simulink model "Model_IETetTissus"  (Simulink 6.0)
settings: Solver=ode45  StartTime=0  StopTime=7E-3  RelTol=1e-3
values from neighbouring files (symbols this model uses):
  b = S/Sm    (= 0.1)    [Constantes.m]    (also in ConstantesBck.m)
  beta = 0.95    [Constantes.m]    (also in ConstantesBck.m; ResCourV1.m = 1; ResCrV1.m = 1; ResEnerV1.m = 1)
  C = 1    [Constantes.m]    (also in ConstantesBck.m)
  Cdl = 603E-9    (= 6.03e-07)    [Constantes.m]    (also in ConstantesBck.m; ResCourV1.m = 7.313e-07; ResCrV1.m = 7.313e-07; ResEnerV1.m = 7.313e-07)
  Cmem = 1E-6*Sm*(1-b)    (= 2.826e-08)    [Constantes.m]    (also in ConstantesBck.m = 3.14e-11; ImpedanceZtissus.m = 4e-08; Ztissus.m = 4e-08; CalculCharge.m = 1)
  gk = 36    [Constantes.m]    (also in ConstantesBck.m; sim_hh.m)
  gl = 0.3    [Constantes.m]    (also in ConstantesBck.m; sim_hh.m)
  gna = 120    [Constantes.m]    (also in ConstantesBck.m; sim_hh.m)
  h0 = 0.5961    [Constantes.m]    (also in ConstantesBck.m)
  m0 = 0.0529    [Constantes.m]    (also in ConstantesBck.m)
  mK = 0    [Constantes.m]    (also in ConstantesBck.m)
  mL = 0    [Constantes.m]    (also in ConstantesBck.m)
  mNa = 0    [Constantes.m]    (also in ConstantesBck.m)
  n0 = 0.3177    [Constantes.m]    (also in ConstantesBck.m)
  rapportIE = 10    [Constantes.m]
  Rcan = 6.398E3*Sm*(1-b)    (= 180.80748)    [Constantes.m]    (also in ConstantesBck.m = 0.03454; ImpedanceZtissus.m = 44; Ztissus.m = 44)
  Rct = 185.6E3    (= 185600)    [Constantes.m]    (also in ConstantesBck.m; ResCourV1.m = 605200; ResCrV1.m = 605200; ResEnerV1.m = 605200)
  Rext = 2.9E3    (= 2900)    [Constantes.m]    (also in ConstantesBck.m)
  Rint = 2.9E2    (= 290)    [Constantes.m]    (also in ConstantesBck.m = 400)
  sigma = 66466    [Constantes.m]    (also in ConstantesBck.m; ResCourV1.m = 68000; ResCrV1.m = 68000; ResEnerV1.m = 68000)
  Sm = 3.14e-2    (= 0.0314)    [Constantes.m]    (also in ConstantesBck.m = 0.000314)
  t0 = 2E-3    (= 0.002)    [Constantes.m]    (also in ConstantesBck.m = 0.001)
  Vk = -82    [Constantes.m]    (also in ConstantesBck.m)
  Vl = -59    [Constantes.m]    (also in ConstantesBck.m)
  Vna = 45    [Constantes.m]    (also in ConstantesBck.m)
  Vr = -70    [Constantes.m]    (also in ConstantesBck.m)
undefined symbols (not defined in the file or in its folder): ln

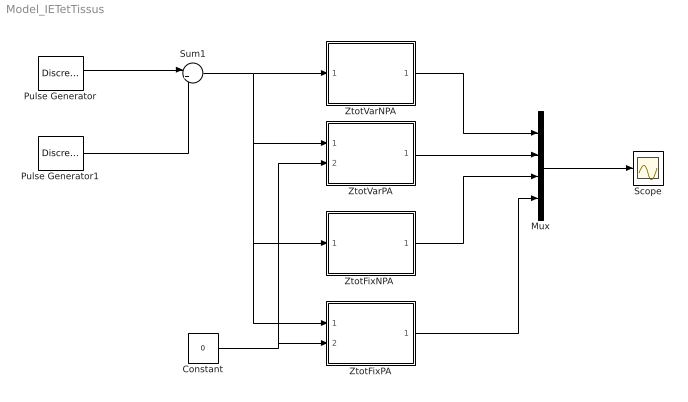
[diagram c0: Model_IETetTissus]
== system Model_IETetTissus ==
  Constant : Constant  Value=0
  Mux : Mux
  Pulse Generator : DiscretePulseGenerator  PulseType=Time based  Amplitude=-160E-6  Period=2*t0  PulseWidth=50  PhaseDelay=t0
  Pulse Generator1 : DiscretePulseGenerator  PulseType=Time based  Amplitude=160E-6  Period=2*t0  PulseWidth=50  PhaseDelay=2*t0
  Scope : Scope
  Sum1 : Sum  Inputs=|++
  "ZtotFixNPA " : Subsystem
  ZtotFixPA : Subsystem
  ZtotVarNPA : Subsystem
  ZtotVarPA : Subsystem
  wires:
  Pulse Generator/1 -> Sum1/1
  Pulse Generator1/1 -> Sum1/2
  Sum1/1 -> ZtotVarNPA/1(InZtot), ZtotVarPA/1(InZtot), "ZtotFixNPA "/1(InZtot), ZtotFixPA/1(InZtot)
  "ZtotFixNPA "/1(OutZtot) -> Mux/3
  ZtotVarPA/1(OutZtot) -> Mux/2
  ZtotFixPA/1(OutZtot) -> Mux/4
  Constant/1 -> ZtotFixPA/2(InVref), ZtotVarPA/2(InVref)
  ZtotVarNPA/1(OutZtot) -> Mux/1
  Mux/1 -> Scope/1

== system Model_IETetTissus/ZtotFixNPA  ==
  InZtot : Inport  Port=1  LatchInput=off
  Gain : Gain
  Sum : Sum  Inputs=|++
  Ziet : Subsystem
  Zmembrane : Subsystem
  OutZtot : Outport
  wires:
  Ziet/1(OutZiet) -> Gain/1
  Zmembrane/1(OutZmem) -> Sum/1
  InZtot/1 -> Zmembrane/1(InZmem), Ziet/1(InZiet)
  Gain/1 -> Sum/2
  Sum/1 -> OutZtot/1

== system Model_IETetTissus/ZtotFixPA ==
  InZtot : Inport  Port=1  LatchInput=off
  InVref : Inport  Port=2  LatchInput=off
  Gain : Gain
  Sum : Sum  Inputs=|++
  ZTissus : Subsystem
  Ziet : Subsystem
  OutZtot : Outport
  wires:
  ZTissus/1(Vout) -> Sum/2
  Ziet/1(OutZiet) -> Gain/1
  InZtot/1 -> ZTissus/1(IStim), Ziet/1(InZiet)
  Sum/1 -> OutZtot/1
  Gain/1 -> Sum/1
  InVref/1 -> ZTissus/2(Vref)

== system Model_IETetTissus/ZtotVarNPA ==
  InZtot : Inport  Port=1  LatchInput=off
  Gain : Gain
  Sum : Sum  Inputs=|++
  ZietVar : Subsystem
  ZmembraneVar : Subsystem
  OutZtot : Outport
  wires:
  ZietVar/1(OutZiet) -> Gain/1
  ZmembraneVar/1(OutZmem) -> Sum/1
  InZtot/1 -> ZmembraneVar/1(InZmem), ZietVar/1(InZiet)
  Gain/1 -> Sum/2
  Sum/1 -> OutZtot/1

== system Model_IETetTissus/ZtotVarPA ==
  InZtot : Inport  Port=1  LatchInput=off
  InVref : Inport  Port=2  LatchInput=off
  Gain : Gain
  Sum : Sum  Inputs=|++
  ZTissusVar : Subsystem
  ZietVar : Subsystem
  OutZtot : Outport
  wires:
  ZietVar/1(OutZiet) -> Gain/1
  ZTissusVar/1(Vout) -> Sum/1
  InZtot/1 -> ZTissusVar/1(IStim), ZietVar/1(InZiet)
  Gain/1 -> Sum/2
  Sum/1 -> OutZtot/1
  InVref/1 -> ZTissusVar/2(Vref)

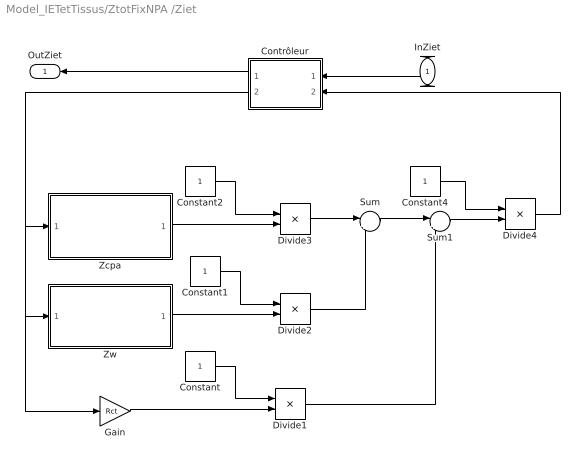
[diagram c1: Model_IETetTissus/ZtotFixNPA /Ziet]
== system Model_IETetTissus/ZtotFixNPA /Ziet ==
  InZiet : Inport  Orientation=left  Port=1  LatchInput=off
  Constant{,1..2,4} (4 alike) : Constant
  Contrôleur : Stateflow chart  Orientation=left
  Divide{1..4} (4 alike) : Product  Inputs=*/  OutScaling=2^-10
  Gain : Gain  Gain=Rct
  Sum : Sum  Inputs=|++
  Sum1 : Sum  Inputs=|++
  Zcpa : Subsystem
  Zw : Subsystem
  OutZiet : Outport  Orientation=left
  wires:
  Constant/1 -> Divide1/1
  Constant1/1 -> Divide2/1
  Constant2/1 -> Divide3/1
  Zcpa/1(OutZcpa) -> Divide3/2
  Zw/1(OutZw) -> Divide2/2
  Divide3/1 -> Sum/1
  Constant4/1 -> Divide4/1
  Divide2/1 -> Sum/2
  Sum/1 -> Sum1/1
  Divide1/1 -> Sum1/2
  Sum1/1 -> Divide4/2
  Divide4/1 -> Contrôleur/2(calc)
  Gain/1 -> Divide1/2
  InZiet/1 -> Contrôleur/1(u)
  Contrôleur/1(y) -> OutZiet/1
  Contrôleur/2(temp) -> Zcpa/1(InZcpa), Zw/1(InZw), Gain/1

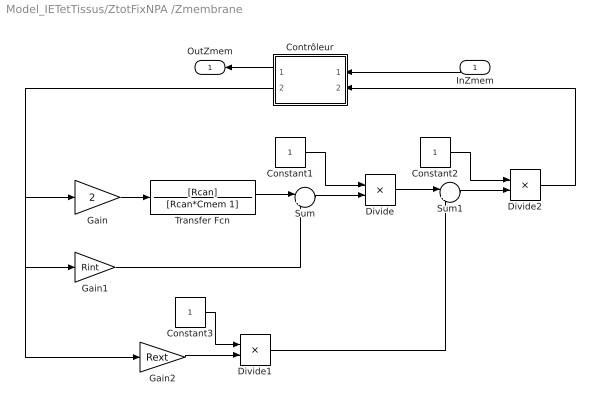
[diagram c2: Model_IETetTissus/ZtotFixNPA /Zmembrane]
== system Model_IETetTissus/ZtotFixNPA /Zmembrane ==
  InZmem : Inport  Orientation=left  Port=1  LatchInput=off
  Constant1 : Constant
  Constant2 : Constant
  Constant3 : Constant
  Contrôleur : Stateflow chart  Orientation=left
  Divide : Product  Inputs=*/  OutScaling=2^-10
  Divide1 : Product  Inputs=*/  OutScaling=2^-10
  Divide2 : Product  Inputs=*/  OutScaling=2^-10
  Gain : Gain  Gain=2
  Gain1 : Gain  Gain=Rint
  Gain2 : Gain  Gain=Rext
  Sum : Sum  Inputs=|++
  Sum1 : Sum  Inputs=|++
  Transfer Fcn : TransferFcn  Numerator=[Rcan]  Denominator=[Rcan*Cmem 1]
  OutZmem : Outport  Orientation=left
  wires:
  Gain/1 -> Transfer Fcn/1
  Transfer Fcn/1 -> Sum/1
  Sum/1 -> Divide/2
  Gain2/1 -> Divide1/2
  Constant1/1 -> Divide/1
  Divide/1 -> Sum1/1
  Constant2/1 -> Divide2/1
  Sum1/1 -> Divide2/2
  Gain1/1 -> Sum/2
  Divide1/1 -> Sum1/2
  Divide2/1 -> Contrôleur/2(calc)
  Constant3/1 -> Divide1/1
  Contrôleur/2(temp) -> Gain2/1, Gain1/1, Gain/1
  InZmem/1 -> Contrôleur/1(u)
  Contrôleur/1(y) -> OutZmem/1

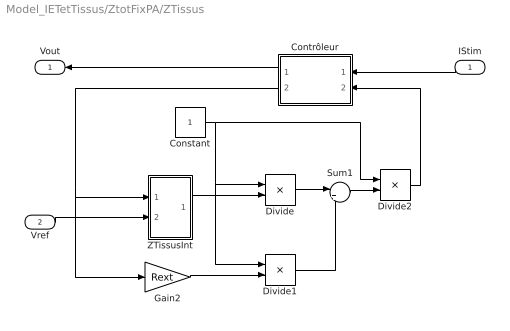
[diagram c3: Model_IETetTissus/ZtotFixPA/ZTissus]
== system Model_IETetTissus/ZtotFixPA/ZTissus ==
  IStim : Inport  Orientation=left  Port=1  LatchInput=off
  Vref : Inport  Port=2  LatchInput=off
  Constant : Constant
  Contrôleur : Stateflow chart  Orientation=left
  Divide : Product  Inputs=*/  OutScaling=2^-10
  Divide1 : Product  Inputs=*/  OutScaling=2^-10
  Divide2 : Product  Inputs=*/  OutScaling=2^-10
  Gain2 : Gain  Gain=Rext
  Sum1 : Sum  Inputs=|++
  ZTissusInt : Subsystem
  Vout : Outport  Orientation=left
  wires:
  Constant/1 -> Divide/1, Divide1/1, Divide2/1
  ZTissusInt/1(Vout) -> Divide/2
  Gain2/1 -> Divide1/2
  Divide/1 -> Sum1/1
  Divide1/1 -> Sum1/2
  Sum1/1 -> Divide2/2
  Vref/1 -> ZTissusInt/2(VRefIn)
  Divide2/1 -> Contrôleur/2(calc)
  Contrôleur/2(temp) -> ZTissusInt/1(InStim), Gain2/1
  IStim/1 -> Contrôleur/1(u)
  Contrôleur/1(y) -> Vout/1

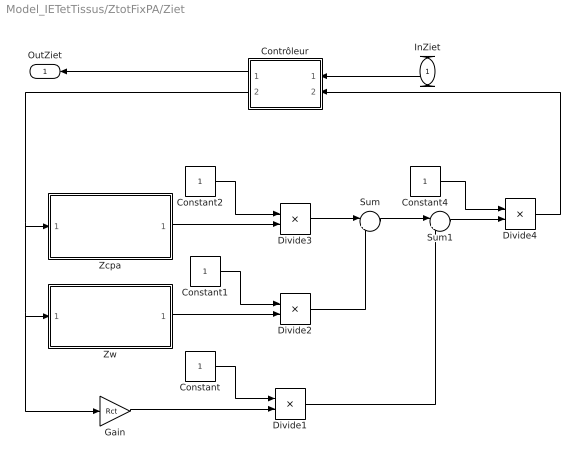
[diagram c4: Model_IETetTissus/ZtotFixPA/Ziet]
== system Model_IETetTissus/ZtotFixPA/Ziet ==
  InZiet : Inport  Orientation=left  Port=1  LatchInput=off
  Constant{,1..2,4} (4 alike) : Constant
  Contrôleur : Stateflow chart  Orientation=left
  Divide{1..4} (4 alike) : Product  Inputs=*/  OutScaling=2^-10
  Gain : Gain  Gain=Rct
  Sum : Sum  Inputs=|++
  Sum1 : Sum  Inputs=|++
  Zcpa : Subsystem
  Zw : Subsystem
  OutZiet : Outport  Orientation=left
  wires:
  Constant/1 -> Divide1/1
  Constant1/1 -> Divide2/1
  Constant2/1 -> Divide3/1
  Zcpa/1(OutZcpa) -> Divide3/2
  Zw/1(OutZw) -> Divide2/2
  Divide3/1 -> Sum/1
  Constant4/1 -> Divide4/1
  Divide2/1 -> Sum/2
  Sum/1 -> Sum1/1
  Divide1/1 -> Sum1/2
  Sum1/1 -> Divide4/2
  Divide4/1 -> Contrôleur/2(calc)
  Gain/1 -> Divide1/2
  InZiet/1 -> Contrôleur/1(u)
  Contrôleur/1(y) -> OutZiet/1
  Contrôleur/2(temp) -> Zcpa/1(InZcpa), Zw/1(InZw), Gain/1

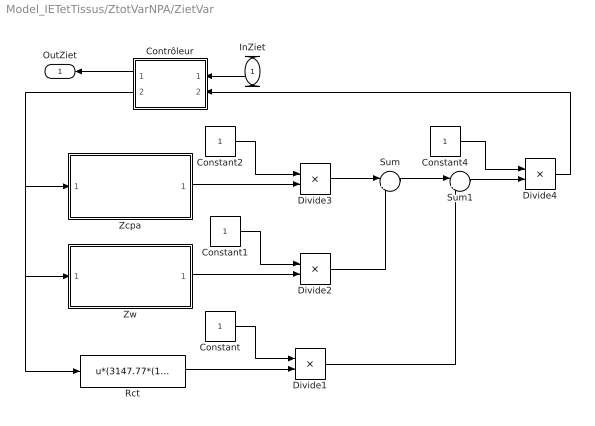
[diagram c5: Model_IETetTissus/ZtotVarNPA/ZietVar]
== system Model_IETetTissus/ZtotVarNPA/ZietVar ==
  InZiet : Inport  Orientation=left  Port=1  LatchInput=off
  Constant{,1..2,4} (4 alike) : Constant
  Contrôleur : Stateflow chart  Orientation=left
  Divide{1..4} (4 alike) : Product  Inputs=*/  OutScaling=2^-10
  Rct : Fcn  Expr=u*(3147.77*(1/((1E6*abs(u))^0.7199)))*1000
  Sum : Sum  Inputs=|++
  Sum1 : Sum  Inputs=|++
  Zcpa : Subsystem
  Zw : Subsystem
  OutZiet : Outport  Orientation=left
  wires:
  Constant/1 -> Divide1/1
  Constant1/1 -> Divide2/1
  Constant2/1 -> Divide3/1
  Zcpa/1(OutZcpa) -> Divide3/2
  Zw/1(OutZw) -> Divide2/2
  Rct/1 -> Divide1/2
  Divide3/1 -> Sum/1
  Constant4/1 -> Divide4/1
  Divide2/1 -> Sum/2
  Sum/1 -> Sum1/1
  Divide1/1 -> Sum1/2
  Sum1/1 -> Divide4/2
  Contrôleur/2(temp) -> Rct/1, Zw/1(InZw), Zcpa/1(InZcpa)
  InZiet/1 -> Contrôleur/1(u)
  Contrôleur/1(y) -> OutZiet/1
  Divide4/1 -> Contrôleur/2(calc)

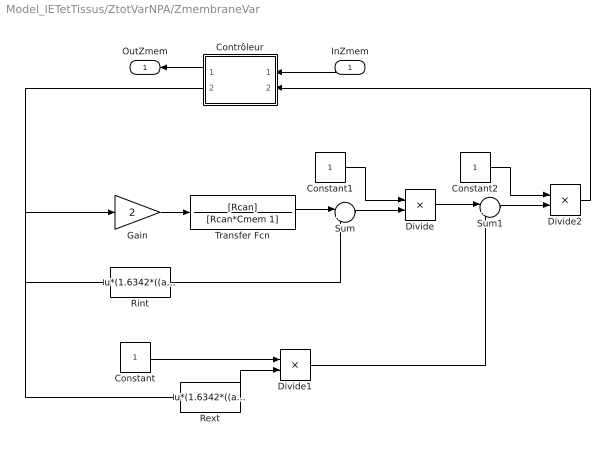
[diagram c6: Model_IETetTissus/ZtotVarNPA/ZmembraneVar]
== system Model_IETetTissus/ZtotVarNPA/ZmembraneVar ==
  InZmem : Inport  Orientation=left  Port=1  LatchInput=off
  Constant : Constant
  Constant1 : Constant
  Constant2 : Constant
  Contrôleur : Stateflow chart  Orientation=left
  Divide : Product  Inputs=*/  OutScaling=2^-10
  Divide1 : Product  Inputs=*/  OutScaling=2^-10
  Divide2 : Product  Inputs=*/  OutScaling=2^-10
  Gain : Gain  Gain=2
  Rext : Fcn  Expr=u*(1.6342*((abs(u)*1E6)^0.1267))*1E3
  Rint : Fcn  Expr=u*(1.6342*((abs(u)*1E6)^0.1267))*1E3/rapportIE
  Sum : Sum  Inputs=|++
  Sum1 : Sum  Inputs=|++
  Transfer Fcn : TransferFcn  Numerator=[Rcan]  Denominator=[Rcan*Cmem 1]
  OutZmem : Outport  Orientation=left
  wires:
  Gain/1 -> Transfer Fcn/1
  Transfer Fcn/1 -> Sum/1
  Sum/1 -> Divide/2
  Rext/1 -> Divide1/2
  Constant1/1 -> Divide/1
  Constant/1 -> Divide1/1
  Divide/1 -> Sum1/1
  Constant2/1 -> Divide2/1
  Sum1/1 -> Divide2/2
  Rint/1 -> Sum/2
  Divide1/1 -> Sum1/2
  Contrôleur/2(temp) -> Rext/1, Rint/1, Gain/1
  Divide2/1 -> Contrôleur/2(calc)
  InZmem/1 -> Contrôleur/1(u)
  Contrôleur/1(y) -> OutZmem/1

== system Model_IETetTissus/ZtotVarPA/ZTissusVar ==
  IStim : Inport  Orientation=left  Port=1  LatchInput=off
  Vref : Inport  Port=2  LatchInput=off
  Constant : Constant
  Contrôleur : Stateflow chart  Orientation=left
  Divide : Product  Inputs=*/  OutScaling=2^-10
  Divide1 : Product  Inputs=*/  OutScaling=2^-10
  Divide2 : Product  Inputs=*/  OutScaling=2^-10
  Rext1 : Fcn  Expr=u*(1.6342*((abs(u)*1E6)^0.1267))*1E3
  Sum1 : Sum  Inputs=|++
  ZTissusInt : Subsystem
  Vout : Outport  Orientation=left
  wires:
  Constant/1 -> Divide/1, Divide1/1, Divide2/1
  ZTissusInt/1(Vout) -> Divide/2
  Rext1/1 -> Divide1/2
  Divide/1 -> Sum1/1
  Divide1/1 -> Sum1/2
  Sum1/1 -> Divide2/2
  Vref/1 -> ZTissusInt/2(VRefIn)
  Divide2/1 -> Contrôleur/2(calc)
  Contrôleur/2(temp) -> Rext1/1, ZTissusInt/1(InStim)
  IStim/1 -> Contrôleur/1(u)
  Contrôleur/1(y) -> Vout/1

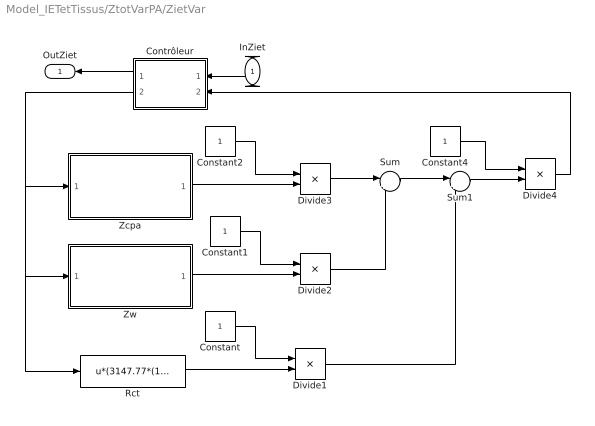
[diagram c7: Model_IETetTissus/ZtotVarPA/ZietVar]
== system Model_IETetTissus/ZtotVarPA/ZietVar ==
  InZiet : Inport  Orientation=left  Port=1  LatchInput=off
  Constant{,1..2,4} (4 alike) : Constant
  Contrôleur : Stateflow chart  Orientation=left
  Divide{1..4} (4 alike) : Product  Inputs=*/  OutScaling=2^-10
  Rct : Fcn  Expr=u*(3147.77*(1/((1E6*abs(u))^0.7199)))*1000
  Sum : Sum  Inputs=|++
  Sum1 : Sum  Inputs=|++
  Zcpa : Subsystem
  Zw : Subsystem
  OutZiet : Outport  Orientation=left
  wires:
  Constant/1 -> Divide1/1
  Constant1/1 -> Divide2/1
  Constant2/1 -> Divide3/1
  Zcpa/1(OutZcpa) -> Divide3/2
  Zw/1(OutZw) -> Divide2/2
  Rct/1 -> Divide1/2
  Divide3/1 -> Sum/1
  Constant4/1 -> Divide4/1
  Divide2/1 -> Sum/2
  Sum/1 -> Sum1/1
  Divide1/1 -> Sum1/2
  Sum1/1 -> Divide4/2
  Contrôleur/2(temp) -> Rct/1, Zw/1(InZw), Zcpa/1(InZcpa)
  InZiet/1 -> Contrôleur/1(u)
  Contrôleur/1(y) -> OutZiet/1
  Divide4/1 -> Contrôleur/2(calc)

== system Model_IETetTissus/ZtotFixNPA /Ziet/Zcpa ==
  InZcpa : Inport  Port=1  LatchInput=off
  Fcn : Fcn  Expr=u^beta
  Transfer Fcn : TransferFcn  Denominator=[Cdl 0]
  OutZcpa : Outport
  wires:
  Transfer Fcn/1 -> Fcn/1
  InZcpa/1 -> Transfer Fcn/1
  Fcn/1 -> OutZcpa/1

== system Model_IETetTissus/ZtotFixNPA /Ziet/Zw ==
  InZw : Inport  Port=1  LatchInput=off
  Gain : Gain  Gain=sigma
  Math Function : Math  Operator=sqrt
  Transfer Fcn : TransferFcn  Numerator=[2]  Denominator=[1 0]
  OutZw : Outport
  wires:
  Transfer Fcn/1 -> Math Function/1
  Math Function/1 -> Gain/1
  Gain/1 -> OutZw/1
  InZw/1 -> Transfer Fcn/1

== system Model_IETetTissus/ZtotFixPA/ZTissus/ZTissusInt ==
  InStim : Inport  Orientation=down  Port=1  LatchInput=off
  VRefIn : Inport  Port=2  LatchInput=off
  Constant : Constant  Value=0
  Gain1 : Gain  Gain=Rint
  Gain2 : Gain  Gain=-1
  Gain3 : Gain  Gain=-1
  Gain4 : Gain  Gain=-1
  Modele HH : Subsystem
  Modele HH1 : Subsystem
  Sum1 : Sum  Inputs=|+++
  Vout : Outport
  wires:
  Modele HH1/1(HHout) -> Gain3/1
  Modele HH/1(HHout) -> Gain4/1
  Gain1/1 -> Sum1/2
  Gain2/1 -> Modele HH/1(HHin)
  InStim/1 -> Gain2/1, Gain1/1, Modele HH1/1(HHin)
  Constant/1 -> Modele HH1/2(VRefIn)
  Sum1/1 -> Vout/1
  VRefIn/1 -> Modele HH/2(VRefIn)
  Gain3/1 -> Sum1/1
  Gain4/1 -> Sum1/3

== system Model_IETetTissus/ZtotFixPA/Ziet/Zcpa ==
  InZcpa : Inport  Port=1  LatchInput=off
  Fcn : Fcn  Expr=u^beta
  Transfer Fcn : TransferFcn  Denominator=[Cdl 0]
  OutZcpa : Outport
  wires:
  Transfer Fcn/1 -> Fcn/1
  InZcpa/1 -> Transfer Fcn/1
  Fcn/1 -> OutZcpa/1

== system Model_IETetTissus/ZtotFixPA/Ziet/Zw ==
  InZw : Inport  Port=1  LatchInput=off
  Gain : Gain  Gain=sigma
  Math Function : Math  Operator=sqrt
  Transfer Fcn : TransferFcn  Numerator=[2]  Denominator=[1 0]
  OutZw : Outport
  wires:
  Transfer Fcn/1 -> Math Function/1
  Math Function/1 -> Gain/1
  Gain/1 -> OutZw/1
  InZw/1 -> Transfer Fcn/1

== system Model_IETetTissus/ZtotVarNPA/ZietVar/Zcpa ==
  InZcpa : Inport  Port=1  LatchInput=off
  Cdl : Fcn  Expr=u*1E9/(918.15-80.854*ln(abs(u)*1E6))
  Fcn : Fcn  Expr=u^beta
  Transfer Fcn : TransferFcn  Denominator=[1 0]
  OutZcpa : Outport
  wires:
  Transfer Fcn/1 -> Fcn/1
  InZcpa/1 -> Cdl/1
  Fcn/1 -> OutZcpa/1
  Cdl/1 -> Transfer Fcn/1

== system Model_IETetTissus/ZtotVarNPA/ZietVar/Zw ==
  InZw : Inport  Port=1  LatchInput=off
  Math Function : Math  Operator=sqrt
  Product : Product
  Transfer Fcn : TransferFcn  Numerator=[2]  Denominator=[1 0]
  sigma : Fcn  Expr=(67202-0.0688*((1E6*abs(u))^2)-11.273*(1E6*abs(u)))
  OutZw : Outport
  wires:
  Transfer Fcn/1 -> Math Function/1
  InZw/1 -> Transfer Fcn/1, sigma/1
  Math Function/1 -> Product/1
  sigma/1 -> Product/2
  Product/1 -> OutZw/1

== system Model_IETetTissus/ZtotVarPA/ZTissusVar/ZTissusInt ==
  InStim : Inport  Orientation=down  Port=1  LatchInput=off
  VRefIn : Inport  Port=2  LatchInput=off
  Constant : Constant  Value=0
  Gain2 : Gain  Gain=-1
  Gain3 : Gain  Gain=-1
  Gain4 : Gain  Gain=-1
  Modele HH : Subsystem
  Modele HH1 : Subsystem
  Rint : Fcn  Expr=u*(1.6342*((abs(u)*1E6)^0.1267))*1E3/rapportIE
  Sum1 : Sum  Inputs=|+++
  Vout : Outport
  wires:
  Modele HH1/1(HHout) -> Gain3/1
  Modele HH/1(HHout) -> Gain4/1
  Rint/1 -> Sum1/2
  Gain2/1 -> Modele HH/1(HHin)
  InStim/1 -> Gain2/1, Rint/1, Modele HH1/1(HHin)
  Constant/1 -> Modele HH1/2(VRefIn)
  Sum1/1 -> Vout/1
  VRefIn/1 -> Modele HH/2(VRefIn)
  Gain3/1 -> Sum1/1
  Gain4/1 -> Sum1/3

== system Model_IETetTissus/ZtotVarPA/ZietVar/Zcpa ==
  InZcpa : Inport  Port=1  LatchInput=off
  Cdl : Fcn  Expr=u*1E9/(918.15-80.854*ln(abs(u)*1E6))
  Fcn : Fcn  Expr=u^beta
  Transfer Fcn : TransferFcn  Denominator=[1 0]
  OutZcpa : Outport
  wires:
  Transfer Fcn/1 -> Fcn/1
  InZcpa/1 -> Cdl/1
  Fcn/1 -> OutZcpa/1
  Cdl/1 -> Transfer Fcn/1

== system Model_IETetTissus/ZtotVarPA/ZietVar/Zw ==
  InZw : Inport  Port=1  LatchInput=off
  Math Function : Math  Operator=sqrt
  Product : Product
  Transfer Fcn : TransferFcn  Numerator=[2]  Denominator=[1 0]
  sigma : Fcn  Expr=(67202-0.0688*((1E6*abs(u))^2)-11.273*(1E6*abs(u)))
  OutZw : Outport
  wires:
  Transfer Fcn/1 -> Math Function/1
  InZw/1 -> Transfer Fcn/1, sigma/1
  Math Function/1 -> Product/1
  sigma/1 -> Product/2
  Product/1 -> OutZw/1

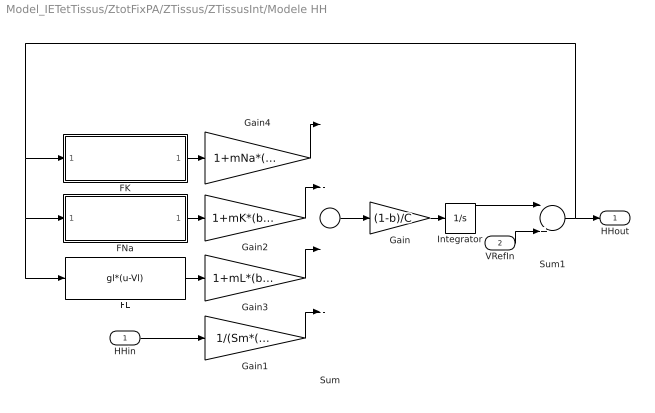
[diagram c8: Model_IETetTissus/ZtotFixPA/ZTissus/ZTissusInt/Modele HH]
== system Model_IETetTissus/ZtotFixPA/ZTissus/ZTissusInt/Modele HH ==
  HHin : Inport  Port=1  LatchInput=off
  VRefIn : Inport  Port=2  LatchInput=off
  FK : Subsystem
  FL : Fcn  Expr=gl*(u-Vl)
  FNa : Subsystem
  Gain : Gain  Gain=(1-b)/C
  Gain1 : Gain  Gain=1/(Sm*(1-b))
  Gain2 : Gain  Gain=1+mK*(b/(1-b))
  Gain3 : Gain  Gain=1+mL*(b/(1-b))
  Gain4 : Gain  Gain=1+mNa*(b/(1-b))
  Integrator : Integrator  InitialCondition=Vr
  Sum : Sum  Inputs=|---+
  Sum1 : Sum  Inputs=|++
  HHout : Outport
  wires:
  Sum/1 -> Gain/1
  Gain/1 -> Integrator/1
  FK/1(FKout) -> Gain4/1
  FNa/1(FNaOut) -> Gain2/1
  FL/1 -> Gain3/1
  HHin/1 -> Gain1/1
  Integrator/1 -> Sum1/1
  Sum1/1 -> HHout/1, FNa/1(FNaIn), FL/1, FK/1(FKIn)
  VRefIn/1 -> Sum1/2
  Gain1/1 -> Sum/4
  Gain4/1 -> Sum/1
  Gain2/1 -> Sum/2
  Gain3/1 -> Sum/3

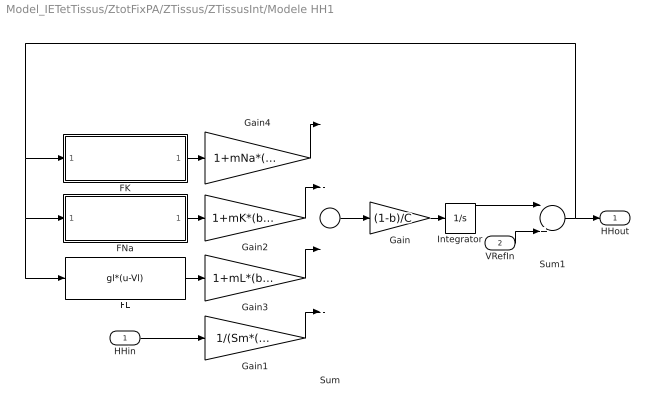
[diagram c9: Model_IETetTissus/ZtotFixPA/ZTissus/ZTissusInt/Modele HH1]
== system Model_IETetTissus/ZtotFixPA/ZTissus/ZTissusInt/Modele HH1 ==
  HHin : Inport  Port=1  LatchInput=off
  VRefIn : Inport  Port=2  LatchInput=off
  FK : Subsystem
  FL : Fcn  Expr=gl*(u-Vl)
  FNa : Subsystem
  Gain : Gain  Gain=(1-b)/C
  Gain1 : Gain  Gain=1/(Sm*(1-b))
  Gain2 : Gain  Gain=1+mK*(b/(1-b))
  Gain3 : Gain  Gain=1+mL*(b/(1-b))
  Gain4 : Gain  Gain=1+mNa*(b/(1-b))
  Integrator : Integrator  InitialCondition=Vr
  Sum : Sum  Inputs=|---+
  Sum1 : Sum  Inputs=|++
  HHout : Outport
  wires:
  Sum/1 -> Gain/1
  Gain/1 -> Integrator/1
  FK/1(FKout) -> Gain4/1
  FNa/1(FNaOut) -> Gain2/1
  FL/1 -> Gain3/1
  HHin/1 -> Gain1/1
  Integrator/1 -> Sum1/1
  Sum1/1 -> HHout/1, FNa/1(FNaIn), FL/1, FK/1(FKIn)
  VRefIn/1 -> Sum1/2
  Gain1/1 -> Sum/4
  Gain4/1 -> Sum/1
  Gain2/1 -> Sum/2
  Gain3/1 -> Sum/3

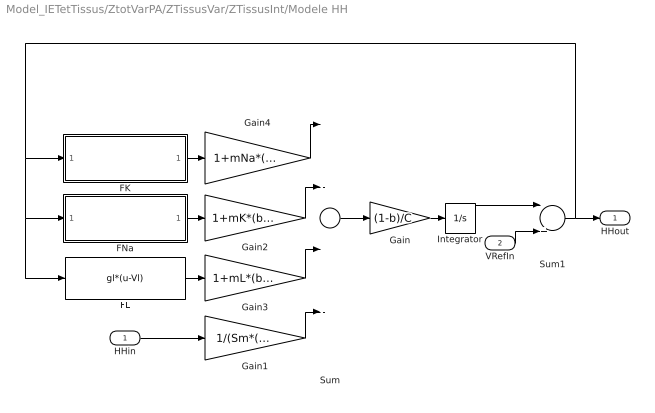
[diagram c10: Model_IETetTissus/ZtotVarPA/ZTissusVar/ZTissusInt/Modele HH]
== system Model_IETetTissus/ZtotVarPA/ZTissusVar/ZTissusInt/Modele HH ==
  HHin : Inport  Port=1  LatchInput=off
  VRefIn : Inport  Port=2  LatchInput=off
  FK : Subsystem
  FL : Fcn  Expr=gl*(u-Vl)
  FNa : Subsystem
  Gain : Gain  Gain=(1-b)/C
  Gain1 : Gain  Gain=1/(Sm*(1-b))
  Gain2 : Gain  Gain=1+mK*(b/(1-b))
  Gain3 : Gain  Gain=1+mL*(b/(1-b))
  Gain4 : Gain  Gain=1+mNa*(b/(1-b))
  Integrator : Integrator  InitialCondition=Vr
  Sum : Sum  Inputs=|---+
  Sum1 : Sum  Inputs=|++
  HHout : Outport
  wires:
  Sum/1 -> Gain/1
  Gain/1 -> Integrator/1
  FK/1(FKout) -> Gain4/1
  FNa/1(FNaOut) -> Gain2/1
  FL/1 -> Gain3/1
  HHin/1 -> Gain1/1
  Integrator/1 -> Sum1/1
  Sum1/1 -> HHout/1, FNa/1(FNaIn), FL/1, FK/1(FKIn)
  VRefIn/1 -> Sum1/2
  Gain1/1 -> Sum/4
  Gain4/1 -> Sum/1
  Gain2/1 -> Sum/2
  Gain3/1 -> Sum/3

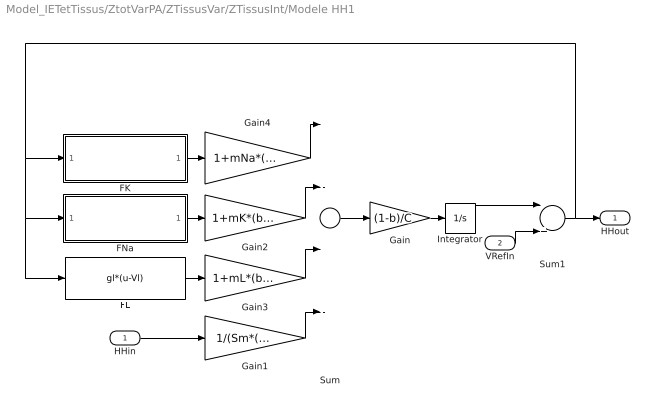
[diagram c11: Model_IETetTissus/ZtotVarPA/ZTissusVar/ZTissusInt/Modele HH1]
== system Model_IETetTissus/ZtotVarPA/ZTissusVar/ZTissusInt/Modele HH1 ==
  HHin : Inport  Port=1  LatchInput=off
  VRefIn : Inport  Port=2  LatchInput=off
  FK : Subsystem
  FL : Fcn  Expr=gl*(u-Vl)
  FNa : Subsystem
  Gain : Gain  Gain=(1-b)/C
  Gain1 : Gain  Gain=1/(Sm*(1-b))
  Gain2 : Gain  Gain=1+mK*(b/(1-b))
  Gain3 : Gain  Gain=1+mL*(b/(1-b))
  Gain4 : Gain  Gain=1+mNa*(b/(1-b))
  Integrator : Integrator  InitialCondition=Vr
  Sum : Sum  Inputs=|---+
  Sum1 : Sum  Inputs=|++
  HHout : Outport
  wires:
  Sum/1 -> Gain/1
  Gain/1 -> Integrator/1
  FK/1(FKout) -> Gain4/1
  FNa/1(FNaOut) -> Gain2/1
  FL/1 -> Gain3/1
  HHin/1 -> Gain1/1
  Integrator/1 -> Sum1/1
  Sum1/1 -> HHout/1, FNa/1(FNaIn), FL/1, FK/1(FKIn)
  VRefIn/1 -> Sum1/2
  Gain1/1 -> Sum/4
  Gain4/1 -> Sum/1
  Gain2/1 -> Sum/2
  Gain3/1 -> Sum/3

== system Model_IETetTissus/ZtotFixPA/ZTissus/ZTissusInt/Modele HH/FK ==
  note: gkm
  note: (Vm-Vk0)
  FKIn : Inport  Port=1  LatchInput=off
  (Vm-Vk0) : Fcn  Expr=(u-Vk)
  Product : Product
  n(Vm) : Subsystem
  n^4 : Fcn  Expr=gk*(u^4)
  FKout : Outport  InitialOutput=0
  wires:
  n(Vm)/1(n) -> n^4/1
  (Vm-Vk0)/1 -> Product/2
  Product/1 -> FKout/1
  n^4/1 -> Product/1
  FKIn/1 -> n(Vm)/1(Vm), (Vm-Vk0)/1

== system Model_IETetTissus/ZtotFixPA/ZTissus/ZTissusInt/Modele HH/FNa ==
  note: gNa*m^3
  note: m
  note: h
  note: gNam
  note: (Vm-VNa0)
  FNaIn : Inport  Port=1  LatchInput=off
  (Vm-VNa0) : Fcn  Expr=(u-Vna)
  Product : Product
  Product1 : Product
  gna*m^3 : Fcn  Expr=gna*u^3
  h(Vm) : Subsystem
  m(Vm) : Subsystem
  FNaOut : Outport  InitialOutput=0
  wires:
  (Vm-VNa0)/1 -> Product1/2
  gna*m^3/1 -> Product/1
  Product1/1 -> FNaOut/1
  FNaIn/1 -> m(Vm)/1(Vm), h(Vm)/1(Vm), (Vm-VNa0)/1
  m(Vm)/1(n) -> gna*m^3/1
  h(Vm)/1(h) -> Product/2
  Product/1 -> Product1/1

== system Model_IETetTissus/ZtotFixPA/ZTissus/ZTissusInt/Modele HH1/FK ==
  note: gkm
  note: (Vm-Vk0)
  FKIn : Inport  Port=1  LatchInput=off
  (Vm-Vk0) : Fcn  Expr=(u-Vk)
  Product : Product
  n(Vm) : Subsystem
  n^4 : Fcn  Expr=gk*(u^4)
  FKout : Outport  InitialOutput=0
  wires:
  n(Vm)/1(n) -> n^4/1
  (Vm-Vk0)/1 -> Product/2
  Product/1 -> FKout/1
  n^4/1 -> Product/1
  FKIn/1 -> n(Vm)/1(Vm), (Vm-Vk0)/1

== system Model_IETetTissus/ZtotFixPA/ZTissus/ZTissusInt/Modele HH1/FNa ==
  note: gNa*m^3
  note: m
  note: h
  note: gNam
  note: (Vm-VNa0)
  FNaIn : Inport  Port=1  LatchInput=off
  (Vm-VNa0) : Fcn  Expr=(u-Vna)
  Product : Product
  Product1 : Product
  gna*m^3 : Fcn  Expr=gna*u^3
  h(Vm) : Subsystem
  m(Vm) : Subsystem
  FNaOut : Outport  InitialOutput=0
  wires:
  (Vm-VNa0)/1 -> Product1/2
  gna*m^3/1 -> Product/1
  Product1/1 -> FNaOut/1
  FNaIn/1 -> m(Vm)/1(Vm), h(Vm)/1(Vm), (Vm-VNa0)/1
  m(Vm)/1(n) -> gna*m^3/1
  h(Vm)/1(h) -> Product/2
  Product/1 -> Product1/1

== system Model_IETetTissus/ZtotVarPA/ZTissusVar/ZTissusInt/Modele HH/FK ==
  note: gkm
  note: (Vm-Vk0)
  FKIn : Inport  Port=1  LatchInput=off
  (Vm-Vk0) : Fcn  Expr=(u-Vk)
  Product : Product
  n(Vm) : Subsystem
  n^4 : Fcn  Expr=gk*(u^4)
  FKout : Outport  InitialOutput=0
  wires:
  n(Vm)/1(n) -> n^4/1
  (Vm-Vk0)/1 -> Product/2
  Product/1 -> FKout/1
  n^4/1 -> Product/1
  FKIn/1 -> n(Vm)/1(Vm), (Vm-Vk0)/1

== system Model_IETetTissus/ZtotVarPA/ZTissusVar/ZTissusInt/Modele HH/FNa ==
  note: gNa*m^3
  note: m
  note: h
  note: gNam
  note: (Vm-VNa0)
  FNaIn : Inport  Port=1  LatchInput=off
  (Vm-VNa0) : Fcn  Expr=(u-Vna)
  Product : Product
  Product1 : Product
  gna*m^3 : Fcn  Expr=gna*u^3
  h(Vm) : Subsystem
  m(Vm) : Subsystem
  FNaOut : Outport  InitialOutput=0
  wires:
  (Vm-VNa0)/1 -> Product1/2
  gna*m^3/1 -> Product/1
  Product1/1 -> FNaOut/1
  FNaIn/1 -> m(Vm)/1(Vm), h(Vm)/1(Vm), (Vm-VNa0)/1
  m(Vm)/1(n) -> gna*m^3/1
  h(Vm)/1(h) -> Product/2
  Product/1 -> Product1/1

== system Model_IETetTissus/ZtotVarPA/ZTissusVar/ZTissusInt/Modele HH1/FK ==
  note: gkm
  note: (Vm-Vk0)
  FKIn : Inport  Port=1  LatchInput=off
  (Vm-Vk0) : Fcn  Expr=(u-Vk)
  Product : Product
  n(Vm) : Subsystem
  n^4 : Fcn  Expr=gk*(u^4)
  FKout : Outport  InitialOutput=0
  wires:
  n(Vm)/1(n) -> n^4/1
  (Vm-Vk0)/1 -> Product/2
  Product/1 -> FKout/1
  n^4/1 -> Product/1
  FKIn/1 -> n(Vm)/1(Vm), (Vm-Vk0)/1

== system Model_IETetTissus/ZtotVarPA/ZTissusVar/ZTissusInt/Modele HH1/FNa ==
  note: gNa*m^3
  note: m
  note: h
  note: gNam
  note: (Vm-VNa0)
  FNaIn : Inport  Port=1  LatchInput=off
  (Vm-VNa0) : Fcn  Expr=(u-Vna)
  Product : Product
  Product1 : Product
  gna*m^3 : Fcn  Expr=gna*u^3
  h(Vm) : Subsystem
  m(Vm) : Subsystem
  FNaOut : Outport  InitialOutput=0
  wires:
  (Vm-VNa0)/1 -> Product1/2
  gna*m^3/1 -> Product/1
  Product1/1 -> FNaOut/1
  FNaIn/1 -> m(Vm)/1(Vm), h(Vm)/1(Vm), (Vm-VNa0)/1
  m(Vm)/1(n) -> gna*m^3/1
  h(Vm)/1(h) -> Product/2
  Product/1 -> Product1/1

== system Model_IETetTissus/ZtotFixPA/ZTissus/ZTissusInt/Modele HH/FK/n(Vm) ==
  note: V
  note: alpha_*(1-n)
  note: beta_n*n
  note: n
  note: n
  Vm : Inport  Port=1  LatchInput=off
  (1-n) : Fcn  Expr=1-u
  Integrator1 : Integrator  InitialCondition=n0
  Product : Product
  Product1 : Product
  Sum1 : Sum  Inputs=+-
  V : Fcn  Expr=u-Vr
  alpha_n : Fcn  Expr=(0.01*(10-u))/(exp((10-u)/10)-1)
  beta_n : Fcn  Expr=0.125*exp(-u/80)
  n : Outport  InitialOutput=0
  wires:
  V/1 -> alpha_n/1, beta_n/1
  alpha_n/1 -> Product/2
  (1-n)/1 -> Product/1
  beta_n/1 -> Product1/1
  Product/1 -> Sum1/1
  Product1/1 -> Sum1/2
  Sum1/1 -> Integrator1/1
  Integrator1/1 -> (1-n)/1, Product1/2, n/1
  Vm/1 -> V/1

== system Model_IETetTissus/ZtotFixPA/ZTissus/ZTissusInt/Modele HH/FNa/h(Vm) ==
  note: h
  note: h
  note: beta_h*h
  note: alpha_h*(1-h)
  note: V
  Vm : Inport  Port=1  LatchInput=off
  (1-h) : Fcn  Expr=1-u
  Integrator1 : Integrator  InitialCondition=h0
  Product : Product
  Product1 : Product
  Sum1 : Sum  Inputs=+-
  V : Fcn  Expr=u-Vr
  alpha_h : Fcn  Expr=0.07*exp(-u/20)
  beta_h : Fcn  Expr=1/(exp((30-u)/10)+1)
  h : Outport  InitialOutput=0
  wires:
  Vm/1 -> V/1
  Integrator1/1 -> h/1, Product1/2, (1-h)/1
  Sum1/1 -> Integrator1/1
  Product1/1 -> Sum1/2
  Product/1 -> Sum1/1
  beta_h/1 -> Product1/1
  (1-h)/1 -> Product/1
  alpha_h/1 -> Product/2
  V/1 -> beta_h/1, alpha_h/1

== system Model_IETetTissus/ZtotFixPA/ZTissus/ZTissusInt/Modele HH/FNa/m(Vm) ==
  note: m
  note: m
  note: beta_m*m
  note: alpha_m*(1-m)
  note: V
  Vm : Inport  Port=1  LatchInput=off
  (1-m) : Fcn  Expr=1-u
  Integrator1 : Integrator  InitialCondition=m0
  Product : Product
  Product1 : Product
  Sum1 : Sum  Inputs=+-
  V : Fcn  Expr=u-Vr
  alpha_m : Fcn  Expr=(0.1*(25-u))/(exp((25-u)/10)-1)
  beta_m : Fcn  Expr=4*exp(-u/18)
  n : Outport  InitialOutput=0
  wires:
  Vm/1 -> V/1
  Integrator1/1 -> n/1, Product1/2, (1-m)/1
  Sum1/1 -> Integrator1/1
  Product1/1 -> Sum1/2
  Product/1 -> Sum1/1
  beta_m/1 -> Product1/1
  (1-m)/1 -> Product/1
  alpha_m/1 -> Product/2
  V/1 -> beta_m/1, alpha_m/1

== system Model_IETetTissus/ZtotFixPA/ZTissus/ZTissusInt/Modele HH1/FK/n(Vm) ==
  note: V
  note: alpha_*(1-n)
  note: beta_n*n
  note: n
  note: n
  Vm : Inport  Port=1  LatchInput=off
  (1-n) : Fcn  Expr=1-u
  Integrator1 : Integrator  InitialCondition=n0
  Product : Product
  Product1 : Product
  Sum1 : Sum  Inputs=+-
  V : Fcn  Expr=u-Vr
  alpha_n : Fcn  Expr=(0.01*(10-u))/(exp((10-u)/10)-1)
  beta_n : Fcn  Expr=0.125*exp(-u/80)
  n : Outport  InitialOutput=0
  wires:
  V/1 -> alpha_n/1, beta_n/1
  alpha_n/1 -> Product/2
  (1-n)/1 -> Product/1
  beta_n/1 -> Product1/1
  Product/1 -> Sum1/1
  Product1/1 -> Sum1/2
  Sum1/1 -> Integrator1/1
  Integrator1/1 -> (1-n)/1, Product1/2, n/1
  Vm/1 -> V/1

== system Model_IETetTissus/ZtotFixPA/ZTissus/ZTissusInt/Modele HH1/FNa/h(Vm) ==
  note: h
  note: h
  note: beta_h*h
  note: alpha_h*(1-h)
  note: V
  Vm : Inport  Port=1  LatchInput=off
  (1-h) : Fcn  Expr=1-u
  Integrator1 : Integrator  InitialCondition=h0
  Product : Product
  Product1 : Product
  Sum1 : Sum  Inputs=+-
  V : Fcn  Expr=u-Vr
  alpha_h : Fcn  Expr=0.07*exp(-u/20)
  beta_h : Fcn  Expr=1/(exp((30-u)/10)+1)
  h : Outport  InitialOutput=0
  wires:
  Vm/1 -> V/1
  Integrator1/1 -> h/1, Product1/2, (1-h)/1
  Sum1/1 -> Integrator1/1
  Product1/1 -> Sum1/2
  Product/1 -> Sum1/1
  beta_h/1 -> Product1/1
  (1-h)/1 -> Product/1
  alpha_h/1 -> Product/2
  V/1 -> beta_h/1, alpha_h/1

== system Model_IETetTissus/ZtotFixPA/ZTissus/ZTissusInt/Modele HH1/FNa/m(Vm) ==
  note: m
  note: m
  note: beta_m*m
  note: alpha_m*(1-m)
  note: V
  Vm : Inport  Port=1  LatchInput=off
  (1-m) : Fcn  Expr=1-u
  Integrator1 : Integrator  InitialCondition=m0
  Product : Product
  Product1 : Product
  Sum1 : Sum  Inputs=+-
  V : Fcn  Expr=u-Vr
  alpha_m : Fcn  Expr=(0.1*(25-u))/(exp((25-u)/10)-1)
  beta_m : Fcn  Expr=4*exp(-u/18)
  n : Outport  InitialOutput=0
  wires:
  Vm/1 -> V/1
  Integrator1/1 -> n/1, Product1/2, (1-m)/1
  Sum1/1 -> Integrator1/1
  Product1/1 -> Sum1/2
  Product/1 -> Sum1/1
  beta_m/1 -> Product1/1
  (1-m)/1 -> Product/1
  alpha_m/1 -> Product/2
  V/1 -> beta_m/1, alpha_m/1

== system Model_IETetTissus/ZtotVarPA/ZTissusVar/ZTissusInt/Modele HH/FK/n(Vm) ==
  note: V
  note: alpha_*(1-n)
  note: beta_n*n
  note: n
  note: n
  Vm : Inport  Port=1  LatchInput=off
  (1-n) : Fcn  Expr=1-u
  Integrator1 : Integrator  InitialCondition=n0
  Product : Product
  Product1 : Product
  Sum1 : Sum  Inputs=+-
  V : Fcn  Expr=u-Vr
  alpha_n : Fcn  Expr=(0.01*(10-u))/(exp((10-u)/10)-1)
  beta_n : Fcn  Expr=0.125*exp(-u/80)
  n : Outport  InitialOutput=0
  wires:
  V/1 -> alpha_n/1, beta_n/1
  alpha_n/1 -> Product/2
  (1-n)/1 -> Product/1
  beta_n/1 -> Product1/1
  Product/1 -> Sum1/1
  Product1/1 -> Sum1/2
  Sum1/1 -> Integrator1/1
  Integrator1/1 -> (1-n)/1, Product1/2, n/1
  Vm/1 -> V/1

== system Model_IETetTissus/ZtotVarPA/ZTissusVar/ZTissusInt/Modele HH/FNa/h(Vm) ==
  note: h
  note: h
  note: beta_h*h
  note: alpha_h*(1-h)
  note: V
  Vm : Inport  Port=1  LatchInput=off
  (1-h) : Fcn  Expr=1-u
  Integrator1 : Integrator  InitialCondition=h0
  Product : Product
  Product1 : Product
  Sum1 : Sum  Inputs=+-
  V : Fcn  Expr=u-Vr
  alpha_h : Fcn  Expr=0.07*exp(-u/20)
  beta_h : Fcn  Expr=1/(exp((30-u)/10)+1)
  h : Outport  InitialOutput=0
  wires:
  Vm/1 -> V/1
  Integrator1/1 -> h/1, Product1/2, (1-h)/1
  Sum1/1 -> Integrator1/1
  Product1/1 -> Sum1/2
  Product/1 -> Sum1/1
  beta_h/1 -> Product1/1
  (1-h)/1 -> Product/1
  alpha_h/1 -> Product/2
  V/1 -> beta_h/1, alpha_h/1

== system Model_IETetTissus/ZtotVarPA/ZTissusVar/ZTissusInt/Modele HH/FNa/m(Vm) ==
  note: m
  note: m
  note: beta_m*m
  note: alpha_m*(1-m)
  note: V
  Vm : Inport  Port=1  LatchInput=off
  (1-m) : Fcn  Expr=1-u
  Integrator1 : Integrator  InitialCondition=m0
  Product : Product
  Product1 : Product
  Sum1 : Sum  Inputs=+-
  V : Fcn  Expr=u-Vr
  alpha_m : Fcn  Expr=(0.1*(25-u))/(exp((25-u)/10)-1)
  beta_m : Fcn  Expr=4*exp(-u/18)
  n : Outport  InitialOutput=0
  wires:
  Vm/1 -> V/1
  Integrator1/1 -> n/1, Product1/2, (1-m)/1
  Sum1/1 -> Integrator1/1
  Product1/1 -> Sum1/2
  Product/1 -> Sum1/1
  beta_m/1 -> Product1/1
  (1-m)/1 -> Product/1
  alpha_m/1 -> Product/2
  V/1 -> beta_m/1, alpha_m/1

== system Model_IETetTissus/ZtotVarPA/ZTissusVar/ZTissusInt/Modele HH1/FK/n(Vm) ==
  note: V
  note: alpha_*(1-n)
  note: beta_n*n
  note: n
  note: n
  Vm : Inport  Port=1  LatchInput=off
  (1-n) : Fcn  Expr=1-u
  Integrator1 : Integrator  InitialCondition=n0
  Product : Product
  Product1 : Product
  Sum1 : Sum  Inputs=+-
  V : Fcn  Expr=u-Vr
  alpha_n : Fcn  Expr=(0.01*(10-u))/(exp((10-u)/10)-1)
  beta_n : Fcn  Expr=0.125*exp(-u/80)
  n : Outport  InitialOutput=0
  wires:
  V/1 -> alpha_n/1, beta_n/1
  alpha_n/1 -> Product/2
  (1-n)/1 -> Product/1
  beta_n/1 -> Product1/1
  Product/1 -> Sum1/1
  Product1/1 -> Sum1/2
  Sum1/1 -> Integrator1/1
  Integrator1/1 -> (1-n)/1, Product1/2, n/1
  Vm/1 -> V/1

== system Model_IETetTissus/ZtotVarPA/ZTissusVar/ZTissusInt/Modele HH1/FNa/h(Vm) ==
  note: h
  note: h
  note: beta_h*h
  note: alpha_h*(1-h)
  note: V
  Vm : Inport  Port=1  LatchInput=off
  (1-h) : Fcn  Expr=1-u
  Integrator1 : Integrator  InitialCondition=h0
  Product : Product
  Product1 : Product
  Sum1 : Sum  Inputs=+-
  V : Fcn  Expr=u-Vr
  alpha_h : Fcn  Expr=0.07*exp(-u/20)
  beta_h : Fcn  Expr=1/(exp((30-u)/10)+1)
  h : Outport  InitialOutput=0
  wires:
  Vm/1 -> V/1
  Integrator1/1 -> h/1, Product1/2, (1-h)/1
  Sum1/1 -> Integrator1/1
  Product1/1 -> Sum1/2
  Product/1 -> Sum1/1
  beta_h/1 -> Product1/1
  (1-h)/1 -> Product/1
  alpha_h/1 -> Product/2
  V/1 -> beta_h/1, alpha_h/1

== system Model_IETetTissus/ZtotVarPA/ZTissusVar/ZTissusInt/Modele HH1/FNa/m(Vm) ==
  note: m
  note: m
  note: beta_m*m
  note: alpha_m*(1-m)
  note: V
  Vm : Inport  Port=1  LatchInput=off
  (1-m) : Fcn  Expr=1-u
  Integrator1 : Integrator  InitialCondition=m0
  Product : Product
  Product1 : Product
  Sum1 : Sum  Inputs=+-
  V : Fcn  Expr=u-Vr
  alpha_m : Fcn  Expr=(0.1*(25-u))/(exp((25-u)/10)-1)
  beta_m : Fcn  Expr=4*exp(-u/18)
  n : Outport  InitialOutput=0
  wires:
  Vm/1 -> V/1
  Integrator1/1 -> n/1, Product1/2, (1-m)/1
  Sum1/1 -> Integrator1/1
  Product1/1 -> Sum1/2
  Product/1 -> Sum1/1
  beta_m/1 -> Product1/1
  (1-m)/1 -> Product/1
  alpha_m/1 -> Product/2
  V/1 -> beta_m/1, alpha_m/1

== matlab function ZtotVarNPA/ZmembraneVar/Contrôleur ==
function [y,temp] = fcn(u,calc)
% This block supports an embeddable subset of the MATLAB language.
% See the help menu for details. 

if u == 0
    y = 0;
    temp = 1E-6;
else
    y = calc;
    temp = u;
end

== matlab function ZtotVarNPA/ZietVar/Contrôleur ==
function [y,temp] = fcn(u,calc)
% This block supports an embeddable subset of the MATLAB language.
% See the help menu for details. 

if u == 0
    y = 0;
    temp = 1E-6;
else
    y = calc;
    temp = u;
end

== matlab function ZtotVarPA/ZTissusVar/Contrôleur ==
function [y,temp] = fcn(u,calc)
% This block supports an embeddable subset of the MATLAB language.
% See the help menu for details. 

if u == 0
    y = 0;
    temp = 1E-6;
else
    y = calc;
    temp = u;
end

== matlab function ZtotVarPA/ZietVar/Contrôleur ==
function [y,temp] = fcn(u,calc)
% This block supports an embeddable subset of the MATLAB language.
% See the help menu for details. 

if u == 0
    y = 0;
    temp = 1E-6;
else
    y = calc;
    temp = u;
end

== matlab function ZtotFixNPA
/Zmembrane/Contrôleur ==
function [y,temp] = fcn(u,calc)
% This block supports an embeddable subset of the MATLAB language.
% See the help menu for details. 

if u == 0
    y = 0;
    temp = 1E-6;
else
    y = calc;
    temp = u;
end

== matlab function ZtotFixNPA
/Ziet/Contrôleur ==
function [y,temp] = fcn(u,calc)
% This block supports an embeddable subset of the MATLAB language.
% See the help menu for details. 

if u == 0
    y = 0;
    temp = 1E-6;
else
    y = calc;
    temp = u;
end

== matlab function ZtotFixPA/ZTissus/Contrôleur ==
function [y,temp] = fcn(u,calc)
% This block supports an embeddable subset of the MATLAB language.
% See the help menu for details. 

if u == 0
    y = 0;
    temp = 1E-6;
else
    y = calc;
    temp = u;
end

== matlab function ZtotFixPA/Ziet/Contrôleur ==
function [y,temp] = fcn(u,calc)
% This block supports an embeddable subset of the MATLAB language.
% See the help menu for details. 

if u == 0
    y = 0;
    temp = 1E-6;
else
    y = calc;
    temp = u;
end
